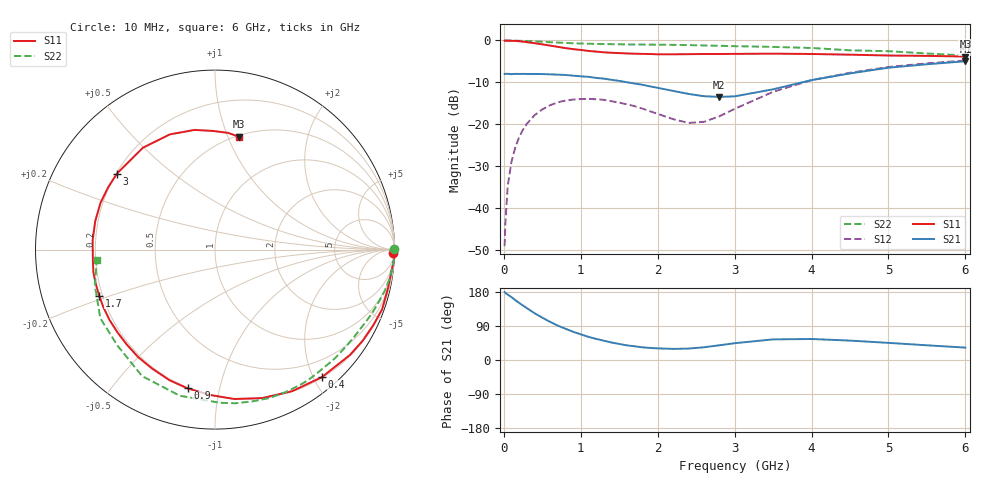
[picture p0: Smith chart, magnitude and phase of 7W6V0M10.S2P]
! Infineon Technologies  Discrete & RF Semiconductors
! BFS17W
! Si NPN RF Bipolar Junction Transistor in SOT323
! VCE = 6 V  IC = 0.1 mA
! Common Emitter S-Parameters:  August  1999
# GHz  S  MA  R  50
!  f  S11  S21  S12  S22
! GHz  MAG  ANG  MAG  ANG  MAG  ANG  MAG  ANG
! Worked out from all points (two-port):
!   36 points, 10 MHz to 6 GHz, reference 50 ohm
!   highest |S21| = -4.97 dB at 6 GHz (marker M1); lowest = -13.5 dB at 2.8 GHz (marker M2)
!   |S21| within 3 dB of the highest: 28.45 MHz to 58.95 MHz (30.5 MHz wide, 69.8 % of centre); 4.468 GHz to end of sweep
!   lowest |S11| = -3.8 dB at 6 GHz (marker M3), VSWR 4.60, Z = 25.7 + j55 ohm
!   |S11| at or under -10 dB: nowhere
!   |S22| runs from -3.6 to 0.0 dB; largest |S21 - S12| = 0.4
!   S11 on the Smith chart (normalised r, x): 10 MHz: 25, -89; 400 MHz: 0.21, -2.13; 900 MHz: 0.20, -0.80; 1.7 GHz: 0.19, -0.19; 3 GHz: 0.20, +0.33; 6 GHz: 0.51, +1.10
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0.01  0.9942 -1.2  0.398 179.3  0.0035 86.2  0.9999 0.2
0.02  0.9999 -2.8  0.399 177.0  0.0065 88.2  0.9911 -0.6
0.05  0.9913 -6.4  0.4 172.8  0.0182 87.9  0.9986 -1.7
0.1  0.9875 -12.5  0.396 165.7  0.0359 82.0  0.9983 -3.5
0.2  0.9774 -25.5  0.398 150.5  0.0705 73.9  0.9908 -6.9
0.3  0.9539 -38.0  0.398 136.7  0.1014 66.0  0.9839 -10.1
0.4  0.9272 -50.0  0.398 123.4  0.1283 58.4  0.9741 -13.4
0.6  0.8683 -72.3  0.394 100.7  0.1682 45.3  0.953 -19.1
0.9  0.7881 -101.2  0.38 74.5  0.1969 29.9  0.9257 -27.4
1.1  0.7496 -117.9  0.368 61.0  0.2008 21.9  0.9143 -32.7
1.4  0.7126 -139.7  0.339 46.1  0.1882 13.0  0.9029 -40.7
1.7  0.6946 -158.3  0.306 36.2  0.1643 8.9  0.8935 -49.3
2.2  0.6838 175.6  0.25 29.3  0.1149 18.4  0.8861 -63.8
2.4  0.6858 166.6  0.23 30.2  0.1036 30.9  0.8805 -70.0
2.8  0.6891 149.8  0.212 38.8  0.1241 59.6  0.8638 -82.3
3  0.6913 142.2  0.215 44.3  0.1524 67.5  0.8543 -88.0
3.5  0.6953 125.3  0.261 54.4  0.2436 71.3  0.8375 -103.5
4  0.6894 111.4  0.336 55.4  0.3364 65.3  0.8134 -120.0
4.5  0.6765 99.7  0.404 51.2  0.4113 57.3  0.7623 -135.5
5  0.661 90.9  0.473 45.2  0.4823 49.4  0.7446 -149.1
5.5  0.6544 83.6  0.52 38.8  0.5328 41.6  0.6989 -163.1
6  0.6427 77.9  0.564 32.7  0.5766 34.7  0.6611 -175.2
